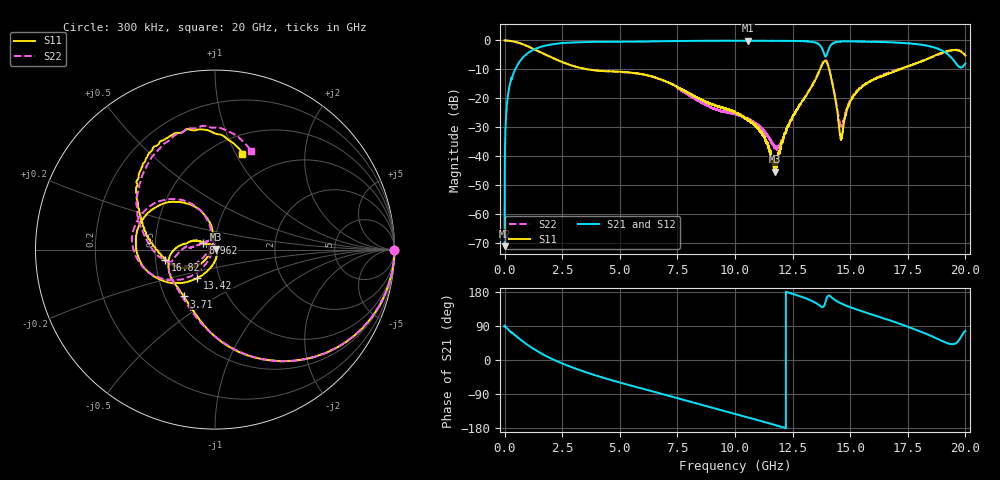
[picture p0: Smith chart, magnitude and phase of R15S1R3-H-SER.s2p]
!{R15S1R3}
!Johanson Technology Inc.
!www.johansontechnology.com
!Test Board Conditions:
!Substrate Type  RO4350B
!Substrate Thickness  20 mil
!Substrate Dk  3.66
!TL Type: GCPW
!TL Trace Width  34 mil
!TL Gap  10 mil
!Electrode orientation  Horizontal
!DUT TOPOLOGY	SERIES
!Mounting Pad LxW  26x52 mil
! Created Sat Feb  6 12:13:09 2021
# hz S ma R 50
! 2 Port Network Data from SP1.SP block
! freq  magS11  angS11  magS21  angS21  magS12  angS12  magS22  angS22
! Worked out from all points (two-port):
!   20001 points, 300 kHz to 20 GHz, reference 50 ohm
!   highest |S21| = -0.09 dB at 10.57 GHz (marker M1); lowest = -70.9 dB at 300 kHz (marker M2)
!   |S21| within 3 dB of the highest: 1.283 GHz to 13.8 GHz (12.52 GHz wide, 166 % of centre); 14.07 GHz to 18.88 GHz (4.814 GHz wide, 29.2 % of centre)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
!   lowest |S11| = -45.3 dB at 11.72 GHz (marker M3), VSWR 1.01, Z = 50.4 + j0.372 ohm
!   |S11| at or under -10 dB: 3.652 GHz to 13.69 GHz (10.04 GHz wide, 116 % of centre); 14.09 GHz to 17.15 GHz (3.061 GHz wide, 19.6 % of centre); 17.15232 GHz to 17.15645 GHz (4.13 MHz wide, 0.0241 % of centre)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
!   |S22| runs from -37.8 to 0.0 dB; largest |S21 - S12| = 0.016
!   S11 on the Smith chart (normalised r, x): 300 kHz: open; 3.71 GHz: 0.62, -0.36; 8.962 GHz: 0.87, +0.07; 13.42 GHz: 0.78, -0.26; 16.82 GHz: 0.56, -0.07; 20 GHz: 0.70, +1.06
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300000  1 -0.2  0.0002844 90.0  0.0001681 82.3  0.9983 -0.2
1.303e8  0.9943 -7.7  0.1021 82.0  0.1027 82.0  0.9937 -7.7
5.013e8  0.9374 -26.6  0.3432 63.1  0.3442 63.2  0.9357 -26.6
1.8273e9  0.5591 -80.2  0.8237 9.6  0.8249 9.6  0.5553 -80.2
3.3343e9  0.334 -116.7  0.937 -28.2  0.9369 -28.2  0.3334 -119.7
3.7103e9  0.3136 -123.8  0.9437 -35.9  0.9437 -35.9  0.3123 -128.0
6.6673e9  0.2209 178.3  0.966 -86.8  0.9672 -86.8  0.2204 -171.0
8.9623e9  0.07999 150.4  0.9879 -125.1  0.9869 -125.1  0.07028 144.8
1.00003e10  0.05753 149.0  0.9869 -142.3  0.9879 -142.3  0.05433 109.5
1.05733e10  0.04147 137.1  0.9897 -151.7  0.9865 -151.7  0.04199 103.8
1.17163e10  0.005451 42.7  0.9856 -171.3  0.9855 -171.3  0.01436 141.3
1.23353e10  0.03446 -73.5  0.9812 177.7  0.9823 177.8  0.0344 -130.2
1.33343e10  0.1624 -117.1  0.9462 156.1  0.9489 156.1  0.1667 -128.7
1.34173e10  0.1865 -121.6  0.9321 153.7  0.9367 153.5  0.1912 -131.5
1.37403e10  0.3492 -151.5  0.7786 141.1  0.7829 140.9  0.3625 -155.6
1.39873e10  0.4166 148.0  0.5684 165.0  0.565 164.6  0.4388 146.9
1.46123e10  0.01968 172.7  0.9594 149.1  0.9592 149.1  0.03373 161.0
1.52073e10  0.1178 -136.3  0.9619 134.7  0.9602 135.1  0.1236 -144.6
1.66673e10  0.2673 -165.8  0.9333 105.5  0.9215 105.5  0.2796 -167.1
1.68233e10  0.2843 -168.8  0.9267 102.5  0.9182 102.4  0.2968 -169.9
1.89153e10  0.6009 134.5  0.6914 52.4  0.6934 52.4  0.5844 133.1
2e10  0.5485 73.9  0.4021 76.6  0.398 77.1  0.5823 69.9
